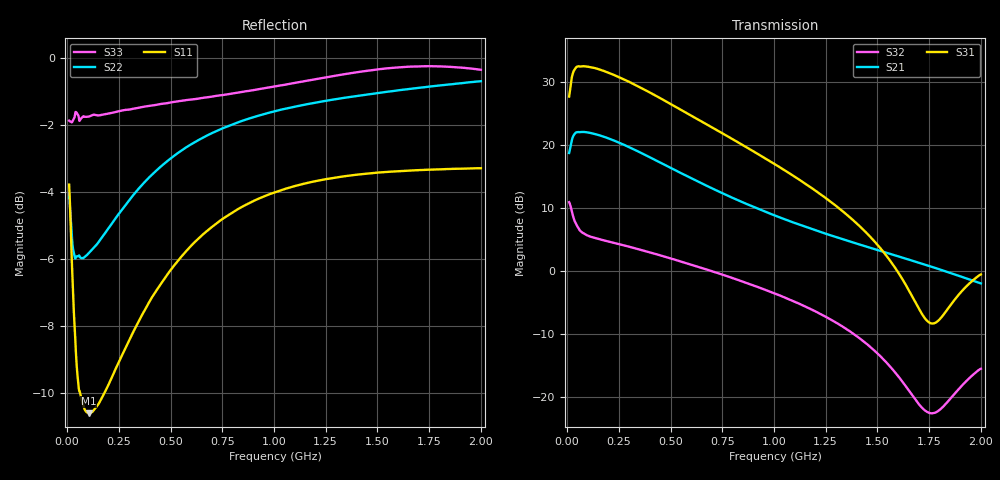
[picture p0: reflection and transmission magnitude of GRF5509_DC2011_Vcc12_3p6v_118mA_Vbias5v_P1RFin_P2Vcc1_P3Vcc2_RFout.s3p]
!Keysight Technologies,N5244B,MY57181157,A.18.40.03
!Date: Wednesday, April 29, 2026 14:28:09
!Correction: S11(C  3-Port  )
!S12(C  3-Port  )
!S13(C  3-Port  )
!S21(C  3-Port  )
!S22(C  3-Port  )
!S23(C  3-Port  )
!S31(C  3-Port  )
!S32(C  3-Port  )
!S33(C  3-Port  )
!S3P File: Measurements: <S11,S12,S13>,
!<S21,S22,S23>,
!<S31,S32,S33>:
# Hz S  dB  R 50
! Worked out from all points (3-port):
!   1991 points, 10 MHz to 2 GHz, reference 50 ohm
!   strongest paths, dB at 10 MHz, 507 MHz, 1.005 GHz, 1.503 GHz, 2 GHz:
!     S31: 27.7, 26.5, 17.0, 4.1, -0.5
!     S21: 18.8, 16.3, 8.9, 3.4, -1.9
!     S32: 11.0, 2.0, -3.5, -13.1, -15.5
!   lowest |S11| = -10.6 dB at 105 MHz (marker M1), VSWR 1.83, Z = 30.9 - j14.9 ohm
!   |S11| at or under -10 dB: 62.54 MHz to 181.3 MHz (118.8 MHz wide, 97.4 % of centre)
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1e7  -3.78 -53.6  -22.19 -33.9  -54.29 -97.2
     18.79 -136.7  -4.03 -78.1  -32.09 -84.1
     27.75 77.7  10.99 -174.2  -1.86 -114.9
3e7  -7.17 -90.0  -26.60 -42.6  -66.35 111.9
     21.48 -161.6  -5.74 -122.1  -43.07 145.8
     31.62 32.2  8.66 161.7  -1.84 -148.9
4.4e7  -8.94 -107.3  -28.64 -42.1  -65.86 -94.9
       22.06 -172.8  -5.94 -136.3  -42.71 -40.1
       32.39 16.0  7.51 158.1  -1.61 -159.1
1.05e8  -10.62 -131.5  -32.32 -31.0  -70.19 42.4
        22.02 163.2  -5.83 -156.3  -50.97 32.0
        32.46 -16.9  5.61 153.8  -1.74 -169.9
1.72e8  -10.11 -137.1  -33.24 -25.3  -68.88 65.4
        21.43 146.1  -5.33 -160.7  -45.36 44.6
        31.87 -38.9  4.97 147.0  -1.68 -172.4
2.52e8  -9.06 -139.2  -33.80 -23.7  -66.21 71.7
        20.42 129.3  -4.64 -163.2  -42.39 42.8
        30.82 -60.0  4.32 137.8  -1.58 -173.2
4.75e8  -6.56 -144.6  -34.86 -25.8  -60.88 87.2
        16.86 95.1  -3.12 -169.9  -39.81 32.7
        27.04 -105.6  2.30 113.3  -1.35 -173.4
6.7e8  -5.20 -150.3  -35.79 -27.8  -58.51 82.5
       13.66 75.4  -2.33 -175.3  -39.33 27.8
       23.42 -135.5  0.35 94.6  -1.17 -173.2
1.005e9  -4.00 -159.3  -37.12 -28.8  -54.91 84.1
         8.86 53.8  -1.58 177.7  -39.93 30.1
         16.99 -175.6  -3.52 66.6  -0.84 -173.4
2e9  -3.29 -178.2  -40.09 -43.9  -48.21 90.8
     -1.91 10.7  -0.68 156.3  -34.87 70.8
     -0.49 -126.3  -15.45 122.3  -0.34 172.2
